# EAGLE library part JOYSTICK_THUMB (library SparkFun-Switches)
Analog Thumb Joystick This is a joystick very similar to the ‘analog’ joysticks on PS2 (PlayStation 2) controllers. Directional movements are simply two potentiometers - one for each axis. Pots are ~10k each. This joystick also has a select button that is actuated when the joystick is pressed down. SparkFun Products Thumb Joystick (COM-09032) SparkFun Thumb Joystick Breakout (BOB-09110) SparkFun Joystick Shield Kit (DEV-09760)
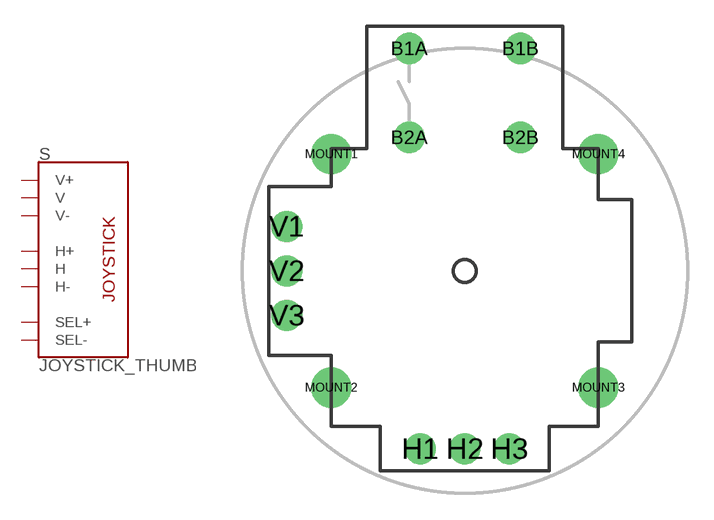
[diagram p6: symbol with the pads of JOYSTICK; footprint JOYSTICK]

Designator prefix S

## JOYSTICK_THUMB (PROD_ID: COMP-09744; SF_SKU: COM-09032)  [JOYSTICK]
B1A  SEL+
B2A  SEL-
H1  H+
H2  H
H3  H-
V1  V+
V2  V
V3  V-

## Footprint JOYSTICK (pad centres in mm)
Thumb Joystick This is a joystick very similar to the ‘analog’ joysticks on PS2 (PlayStation 2) controllers. Directional movements are simply two potentiometers - one for each axis. Pots are ~10k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
drill 0.9 pad 1.778: B1A -3.175,12.7; B1B 3.175,12.7; B2A -3.175,7.62; B2B 3.175,7.62
drill 0.889 pad 1.778: H1 -2.54,-10.16; H2 0,-10.16; H3 2.54,-10.16; V1 -10.16,2.54; V2 -10.16,0; V3 -10.16,-2.54
drill 1.397 pad 2.286: MOUNT1 -7.62,6.668; MOUNT2 -7.62,-6.668; MOUNT3 7.62,-6.668; MOUNT4 7.62,6.668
